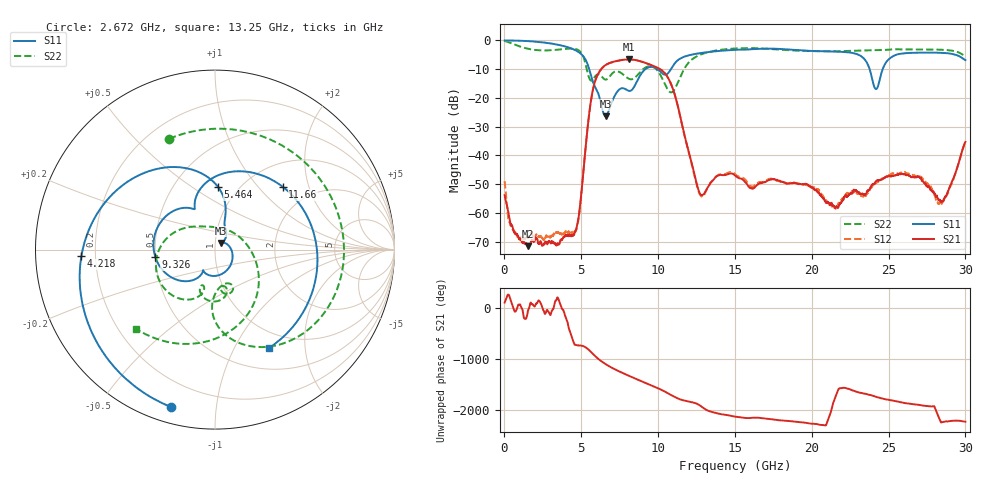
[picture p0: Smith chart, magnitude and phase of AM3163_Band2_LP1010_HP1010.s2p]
!Agilent Technologies,E8364B,MY43040894,A.07.50.67
!Agilent E8364B: A.07.50.67
!Date: Thursday, August 20, 2020 11:15:13
!Correction: S11(Full 2 Port(1,2))
!S21(Full 2 Port(1,2))
!S12(Full 2 Port(1,2))
!S22(Full 2 Port(1,2))
!S2P File: Measurements: S11, S21, S12, S22:
# Hz S  dB  R 50
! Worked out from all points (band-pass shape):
!   3201 points, 10 MHz to 30 GHz, reference 50 ohm
!   highest |S21| = -6.63 dB at 8.079 GHz (marker M1); lowest = -71.6 dB at 1.556 GHz (marker M2)
!   |S21| within 3 dB of the highest: 6.355 GHz to 9.993 GHz (3.638 GHz wide, 44.5 % of centre)
!   lowest |S11| = -26.4 dB at 6.58 GHz (marker M3), VSWR 1.10, Z = 53.1 + j3.88 ohm
!   |S11| at or under -10 dB: 5.514 GHz to 9.173 GHz (3.659 GHz wide, 49.8 % of centre); 9.955 GHz to 10.83 GHz (878.9 MHz wide, 8.46 % of centre); 23.77 GHz to 24.62 GHz (852.5 MHz wide, 3.52 % of centre)
!   |S22| runs from -18.1 to -0.2 dB; largest |S21 - S12| = 0.0034
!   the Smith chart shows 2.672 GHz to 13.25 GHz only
!   S11 on the Smith chart (normalised r, x): 2.672 GHz: 0.07, -0.76; 4.218 GHz: 0.15, -0.02; 5.464 GHz: 0.81, +0.64; 9.326 GHz: 0.50, -0.05; 11.66 GHz: 1.44, +1.37; 13.25 GHz: 0.77, -1.39
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1e7  -0.03 -2.8  -53.82 103.3  -49.00 158.3  -0.22 -8.9
7.035188e8  -0.09 -27.2  -67.34 -74.1  -66.73 -65.4  -1.56 -83.7
1.556359e9  -0.26 -60.7  -71.58 -29.6  -68.45 -42.2  -2.94 -163.6
2.671612e9  -0.81 -105.6  -70.23 -109.9  -68.42 102.3  -3.50 112.5
4.217972e9  -2.55 -177.1  -67.69 -66.8  -66.62 72.0  -2.88 5.7
5.014581e9  -4.86 130.1  -52.65 -22.9  -52.86 -25.2  -4.44 -65.0
5.464431e9  -9.13 87.3  -27.75 -97.9  -27.79 -98.1  -12.31 -89.2
6.579684e9  -26.39 49.5  -8.58 -25.1  -8.61 -25.2  -13.64 -78.0
7.451269e9  -17.19 -69.3  -6.99 -166.2  -7.03 -166.2  -10.93 -98.5
8.079184e9  -17.53 -119.6  -6.63 107.2  -6.65 107.3  -13.30 -111.0
9.325644e9  -9.50 -172.9  -8.14 -53.0  -8.15 -53.1  -9.09 -135.4
1.000979e10  -10.22 133.4  -9.68 -141.9  -9.70 -141.9  -10.84 170.8
1.165924e10  -5.77 42.8  -31.62 -18.5  -31.85 -19.0  -10.32 -36.8
1.325246e10  -4.08 -61.3  -50.96 137.8  -51.02 141.3  -4.12 -134.8
1.5005e10  -3.29 -139.0  -47.01 22.0  -46.46 23.5  -2.83 156.7
1.778845e10  -2.95 96.4  -48.74 -45.4  -48.93 -47.9  -3.18 46.8
2.000958e10  -3.68 -17.0  -51.04 -117.6  -51.31 -113.2  -3.76 -37.5
2.298047e10  -4.86 -140.4  -52.79 145.7  -53.15 146.5  -3.58 -125.2
2.418007e10  -16.93 -147.1  -48.97 52.1  -49.71 57.1  -3.39 -155.4
2.500479e10  -6.61 -132.0  -47.29 -6.6  -46.97 -6.0  -3.26 -175.2
2.837867e10  -4.33 109.2  -55.95 -66.7  -56.35 -107.8  -3.25 97.0
3e10  -6.84 50.3  -35.31 -78.0  -35.56 -78.2  -5.48 48.5
